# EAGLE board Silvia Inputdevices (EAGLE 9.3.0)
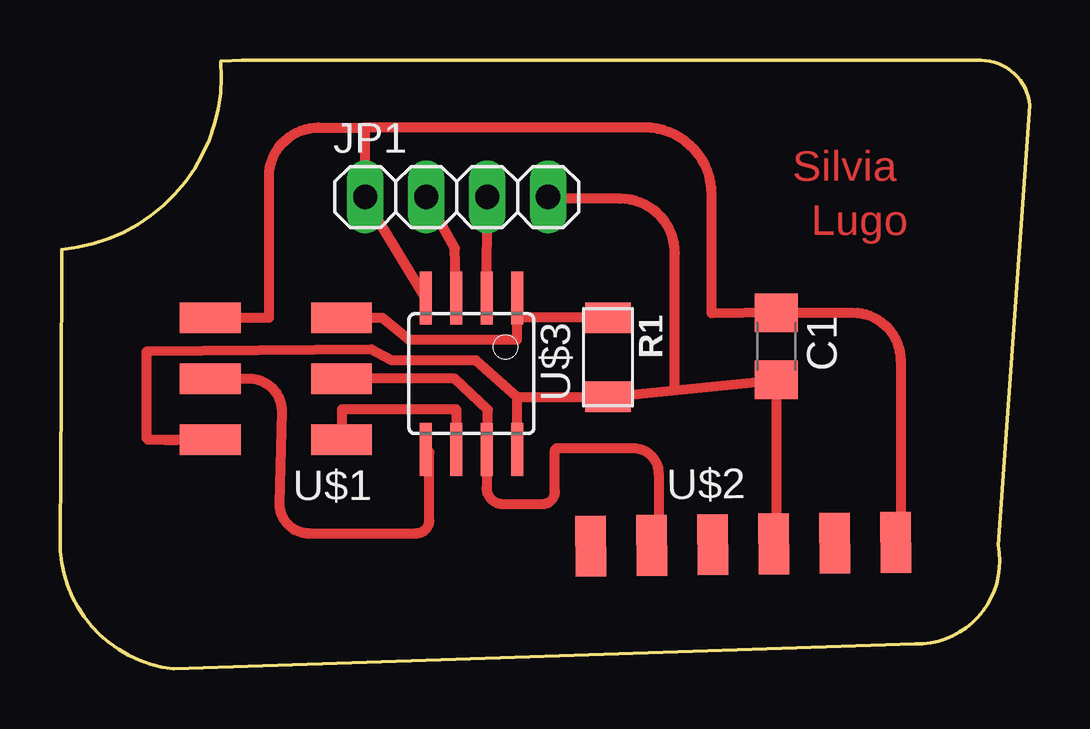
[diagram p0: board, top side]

Size 40.41 x 25.39 mm. Coordinates in mm from the lower left corner, seen from the top.
Outline: 7.59,25.39 6.7,25.34 arc-90 0.07,17.49 0.05,11.4 0,5.41 arc85 4.75,0 35.63,1.04 arc102 39.09,5.16 40.41,23.48 arc85 38.36,25.38 7.59,25.39
Copper layers (1*16): Top 0.035mm / dielectric 1.5mm / Bottom 0.035mm
Design rules "default": minimum track width 10mil, minimum drill 24mil, track to track 8mil, track to pad 8mil, pad to pad 8mil, via to via 8mil, smd to smd 8mil, copper to edge 40mil, drill to drill 8mil, minimum pad ring 10mil, minimum via ring 8mil, stop-mask expansion 4mil, vias tented up to drill 0mil, thermal gap 10mil

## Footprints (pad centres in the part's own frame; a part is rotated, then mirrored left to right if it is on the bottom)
C1206 = smd 1.6 x 1.8: 1 -1.4,0; 2 1.4,0
1X04 = drill 1.016 long: 1 -3.81,0; 2 -1.27,0; 3 1.27,0; 4 3.81,0
R1206FAB = smd 1.27 x 1.905: 1 -1.651,0; 2 1.651,0
2X03SMD = smd 2.54 x 1.27: 1 -2.54,2.54; 2 2.92,2.54; 3 -2.54,0; 4 2.92,0; 5 -2.54,-2.54; 6 2.92,-2.54
1X06SMD = smd 2.54 x 1.27: 1 0,6.35; 2 0,3.81; 3 0,1.27; 4 0,-1.27; 5 0,-3.81; 6 0,-6.35
SOIC8 = smd 0.5 x 2.2: 1 -1.905,-3.154; 2 -0.645,-3.154; 3 0.625,-3.154; 4 1.895,-3.154; 5 1.905,3.154; 6 0.635,3.154; 7 -0.635,3.154; 8 -1.905,3.154

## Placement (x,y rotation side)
C1  CAP-US1206  [C1206]  29.84,13.45 270 top
JP1  [1X04]  16.53,19.68 0 top
R1  10k  [R1206FAB]  22.83,13 270 top
U$1  AVRISPSMD  [2X03SMD]  9.19,12.11 180 top
U$2  FTDI-SMD-HEADER  [1X06SMD]  28.47,5.2 270.7 top
U$3  ATTINY45SI  [SOIC8]  17.14,12.31 180 top

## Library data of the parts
C1 R1 U$1-U$3 = fab
JP1 = pinhead

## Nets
N$1: C1.2 JP1.4 R1.2 U$1.2 U$2.3 U$3.8
N$2: C1.1 JP1.1 U$1.6 U$2.1 U$3.4
N$4: U$1.3 U$2.5 U$3.7
N$5: R1.1 U$1.5 U$3.1
N$6: U$1.1 U$3.6
N$7: U$1.4 U$3.5
N$9: JP1.2 U$3.3
N$10: JP1.3 U$3.2

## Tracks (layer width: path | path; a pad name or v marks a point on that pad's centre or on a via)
N$1
  Top 0.254: 25.32,11.6 25.62,11.63 25.73,11.64 | 29.84,5.31 arc-90 U$2.3 | 3.67,9.55 arc-90 3.6,9.62
  Top 0.406: 4.39,9.54 4.9,9.55 | 4.9,9.55 U$1.2 | 19.04,11.34 19.07,8.27 19.02,8.6 U$3.8 19.04,11.34 | 19.04,11.34 R1.2 | R1.2 23.05,11.32 | 19.04,11.34 17.34,12.87 13.81,12.87 12.97,13.33 3.6,13.22 3.6,9.62 | R1.2 22.62,11.33 25.73,11.64 C1.2 29.84,5.31 | 25.62,11.63 25.62,17.35 arc90 23.36,19.6 20.42,19.6 arc-90 JP1.4 20.34,19.95 arc90 19.83,20.46 | 4.9,9.55 3.67,9.55
N$2
  Top 0.254: 12.72,22.52 arc90 12.67,22.57 | 35.02,5.48 arc-90 U$2.1
  Top 0.406: 6.42,14.62 U$1.6 8.71,14.65 8.71,20.51 arc-90 10.76,22.57 12.67,22.57 24.38,22.57 arc-90 27.15,19.8 27.15,14.82 C1.1 33.04,14.85 arc-90 35.02,12.87 35.02,5.48 | 12.72,22.52 JP1.1 12.72,19.61 U$3.4
N$4
  Top 0.254: 24.94,5.43 arc-90 U$2.5
  Top 0.406: U$1.3 16.45,12.11 17.83,10.81 17.83,9.21 U$3.7 17.77,7.56 arc90 18.46,6.87 20.11,6.87 arc90 20.62,7.38 20.62,9.08 arc-90 20.75,9.21 23.87,9.21 arc-90 24.94,8.14 24.94,5.43
N$5
  Top 0.406: R1.1 19.04,14.65 U$3.1 19.04,13.73 14.55,13.73 13.43,14.65 U$1.5
N$6
  Top 0.406: U$1.1 11.75,10.84 16.5,10.84 U$3.6
N$7
  Top 0.254: 15.39,9.03 arc90 15.26,9.16
  Top 0.406: U$1.4 6.37,12.11 | 15.29,8.25 15.26,9.16 U$3.5 | 5.84,12.11 U$1.4 | 15.39,9.03 15.39,6.19 arc-90 14.85,5.65 10.38,5.65 arc-90 9.14,6.9 9.24,10.73 arc90 7.87,12.11 U$1.4
N$9
  Top 0.406: 16.48,16.55 16.48,15.5 U$3.3 16.45,17.54 JP1.2 15.26,20.72
N$10
  Top 0.406: U$3.2 17.77,15.5 JP1.3 17.8,20.51

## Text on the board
Top: Silvia | Lugo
